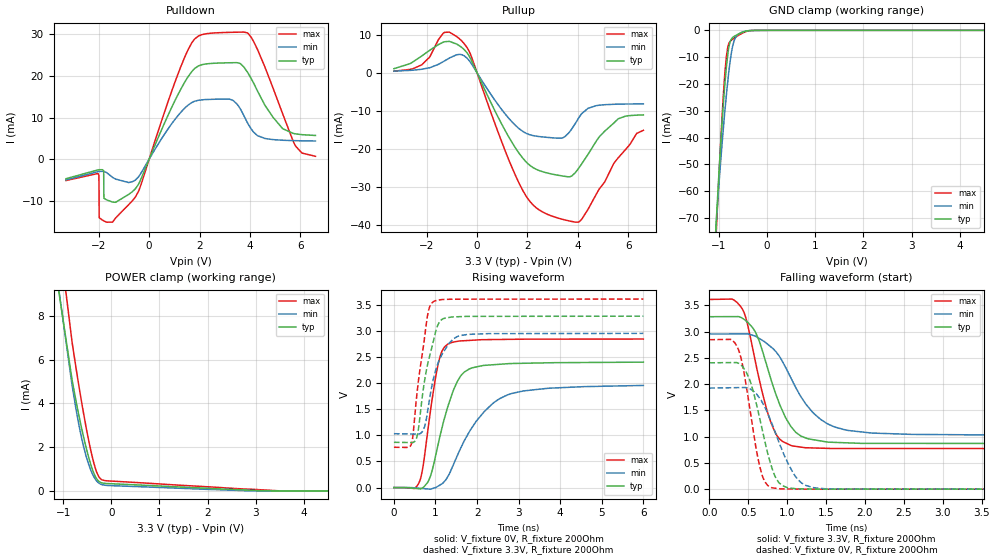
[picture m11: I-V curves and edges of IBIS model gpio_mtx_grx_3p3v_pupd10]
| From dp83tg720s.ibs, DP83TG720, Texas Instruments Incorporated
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| ibis_gtx_mrx_mode10_3p3v
[Model]   gpio_mtx_grx_3p3v_pupd10
Model_type   I/O
Polarity   Non-Inverting
Enable   Active-Low
Vinl = 0.99
Vinh = 2.31
Vmeas = 1.65
Vref = 0
Cref = 2pF
Rref = 100000
|   typ   min   max
C_comp   1.19pF   1.18pF   1.2pF
[Voltage Range]   3.3   2.97   3.63
[Temperature Range]   27   150   -40
[Pullup Reference]   3.3   2.97   3.63
[Pulldown Reference]   0   0   0
[Power Clamp Reference]   3.3   2.97   3.63
[GND Clamp Reference]   0   0   0
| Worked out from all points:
|   slope of the pulldown table from 0 to 0.495 V, typ, clamps not added: 69.8 ohm
|   slope of the pullup table from 0 to 0.495 V, typ, clamps not added: 70 ohm
|   GND clamp passes 1 mA (typ) near -0.55 V on its own axis
|   POWER clamp passes 1 mA (typ) near -0.39 V on its own axis
|   falling waveform, V_fixture 3.3V, R_fixture 200Ohm: 20-80 % time 338ps typ, 481ps min, 270ps max; typ from 3.28 V to 0.868 V
|   rising waveform, V_fixture 0V, R_fixture 200Ohm: 20-80 % time 496ps typ, 912ps min, 312ps max; typ from 0 V to 2.4 V
|   rising waveform, V_fixture 3.3V, R_fixture 200Ohm: 20-80 % time 322ps typ, 369ps min, 266ps max; typ from 0.868 V to 3.28 V
|   falling waveform, V_fixture 0V, R_fixture 200Ohm: 20-80 % time 236ps typ, 329ps min, 190ps max; typ from 2.4 V to 0 V
[Pulldown]
|   Voltage   I(typ)   I(min)   I(max)
-3.3V     -4.691mA   -4.982mA   -5.135mA
-2.033V   -2.58mA    -2.999mA   -3.442mA
-1.993V   -2.544mA   -2.966mA   -3.898mA
-1.983V   -2.536mA   -2.959mA   -14.07mA
-1.795V   -9.393mA   -2.96mA    -14.85mA
-1.449V   -10.32mA   -4.39mA    -15.13mA
-419.1mV  -5.983mA   -4.232mA   -7.676mA
1.541V    19.76mA    12.96mA    26.24mA
2.402V    22.97mA    14.36mA    30.24mA
3.927V    20.65mA    8.469mA    30.21mA
5.808V    6.077mA    4.441mA    3.172mA
6.6V      5.691mA    4.365mA    685.5uA
[GND Clamp]
|   Voltage   I(typ)   I(min)   I(max)
-3.3V     -930.6mA   -801.9mA   -1.027A
-1.132V   -97.01mA   -92.65mA   -104.4mA
-1.053V   -70.04mA   -70.69mA   -73.72mA
-1.043V   -66.78mA   -68.08mA   -69.98mA
-933.9mV  -33.73mA   -41.77mA   -31.53mA
-884.4mV  -21.45mA   -31.4mA    -17.49mA
-844.8mV  -13.41mA   -23.82mA   -9.506mA
-785.4mV  -5.495mA   -13.94mA   -4.56mA
-706.2mV  -2.537mA   -5.166mA   -3.195mA
-646.8mV  -1.864mA   -2.419mA   -2.47mA
-537.9mV  -920uA     -800.8uA   -1.281mA
6.6V      0A         0A         0A
[Pullup]
|   Voltage   I(typ)   I(min)   I(max)
-3.3V     1.091mA    447uA      427.8uA
-2.201V   4.405mA    938uA      2.088mA
-1.29V    8.16mA     3.141mA    10.62mA
-676.5mV  7.008mA    4.855mA    8.806mA
-260.7mV  3.771mA    2.752mA    4.883mA
1.056V    -14.43mA   -10.3mA    -19.45mA
1.818V    -22.43mA   -15.39mA   -30.93mA
2.452V    -25.62mA   -16.72mA   -35.93mA
3.482V    -27.18mA   -16.76mA   -38.61mA
4.135V    -24.07mA   -10.86mA   -38.59mA
5.6V      -12.07mA   -8.226mA   -22.32mA
6.6V      -11.04mA   -8.152mA   -15.09mA
[POWER Clamp]
|   Voltage   I(typ)   I(min)   I(max)
-3.3V     250mA      167.9mA    341.1mA
-1.28V    11.92mA    12.22mA    15.13mA
-815.1mV  5.087mA    4.843mA    6.814mA
-735.9mV  4.149mA    3.783mA    5.67mA
-656.7mV  3.278mA    2.842mA    4.589mA
-518.1mV  1.942mA    1.555mA    2.853mA
-438.9mV  1.302mA    1.024mA    1.985mA
-359.7mV  798.2uA    636.2uA    1.254mA
-300.3mV  544.3uA    443.2uA    841.3uA
-211.2mV  378.3uA    299.6uA    529.3uA
3.482V    0A         0A         5.551uA
6.6V      0A         0A         0A
[Ramp]
R_load = 200
|   typ   min   max
dV/dt_r   1.44153/4.94142e-10   1.17381/9.04282e-10   1.7071/3.1083e-10
dV/dt_f   1.44932/3.38238e-10   1.15335/4.79325e-10   1.70352/2.69155e-10
[Falling Waveform]
V_fixture = 3.3V
V_fixture_min = 2.97V
V_fixture_max = 3.63V
R_fixture = 200Ohm
C_fixture = 0F
|   Time   V(typ)   V(min)   V(max)
0s        3.283V     2.954V     3.612V
289.4ps   3.285V     2.955V     3.619V
424ps     3.254V     2.955V     3.429V
597.2ps   2.976V     2.908V     2.388V
786.9ps   2.112V     2.713V     1.287V
893.6ps   1.652V     2.542V     968mV
1.049ns   1.191V     2.113V     831.6mV
1.355ns   937.3mV    1.424V     783.8mV
1.782ns   881.3mV    1.118V     774.4mV
6ns       867.7mV    1.032V     772.3mV
[Rising Waveform]
V_fixture = 0V
V_fixture_min = 0V
V_fixture_max = 0V
R_fixture = 200Ohm
C_fixture = 0F
|   Time   V(typ)   V(min)   V(max)
0s        398uV      329.9uV    539.7uV
622.6ps   -23.8mV    -13.6mV    129.2mV
707ps     4.019mV    -19.26mV   438.7mV
876.9ps   212.6mV    -30.31mV   1.455V
1.049ns   777.2mV    21.17mV    2.307V
1.294ns   1.546V     207.1mV    2.747V
1.698ns   2.216V     905.3mV    2.814V
2.176ns   2.341V     1.458V     2.834V
2.722ns   2.373V     1.772V     2.839V
6ns       2.403V     1.957V     2.846V
[Rising Waveform]
V_fixture = 3.3V
V_fixture_min = 2.97V
V_fixture_max = 3.63V
R_fixture = 200Ohm
C_fixture = 0F
|   Time   V(typ)   V(min)   V(max)
0s        867.7mV    1.032V     772.3mV
430.2ps   862mV      1.026V     862.4mV
572.8ps   1.037V     1.024V     1.932V
735.2ps   2.036V     1.161V     2.864V
832.5ps   2.437V     1.57V      3.391V
951.6ps   2.814V     2.089V     3.564V
1.138ns   3.211V     2.519V     3.6V
1.339ns   3.261V     2.775V     3.608V
1.587ns   3.275V     2.912V     3.609V
6ns       3.283V     2.954V     3.612V
[Falling Waveform]
|Gnd
V_fixture = 0V
V_fixture_min = 0V
V_fixture_max = 0V
R_fixture = 200Ohm
C_fixture = 0F
|   Time   V(typ)   V(min)   V(max)
0s        2.405V     1.925V     2.846V
274.1ps   2.41V      1.931V     2.852V
370.9ps   2.4V       1.933V     2.667V
514.7ps   2.096V     1.913V     1.586V
642.1ps   1.379V     1.74V      469.2mV
800.8ps   421.5mV    1.262V     28.45mV
894.6ps   121.8mV    893mV      9.11mV
1.089ns   12.02mV    277.9mV    2.674mV
1.355ns   1.707mV    25.54mV    204.7uV
6ns       400.5uV    352.8uV    540.8uV
